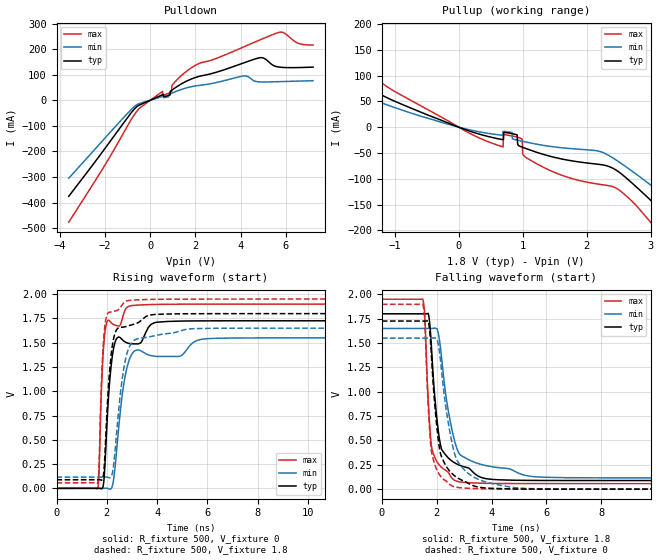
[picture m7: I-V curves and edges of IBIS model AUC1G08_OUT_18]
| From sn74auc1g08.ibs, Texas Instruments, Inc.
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[Model]   AUC1G08_OUT_18
Model_type  Output
Vref =   0
Rref =   1000
Cref =   30p
Vmeas =   0.9
| variable   typ   min   max
C_comp   7.23pF   0.09pF   19.52pF
| C_pullup   7.39pF   0.09pF   19.52pF
| C_pulldown   7.07pF   2.21pF   16.11pF
[Temperature Range]   40   100   -40
| Ambient temperature   25   85   -40
[Voltage range]   1.8   1.65   1.95
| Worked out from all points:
|   slope of the pulldown table from 0 to 0.27 V, typ, clamps not added: 25.5 ohm
|   slope of the pullup table from 0 to 0.27 V, typ, clamps not added: 23.3 ohm
|   rising waveform, R_fixture 500, V_fixture 0: 20-80 % time 284ps typ, 437ps min, 176ps max; typ from 0 V to 1.73 V
|   falling waveform, R_fixture 500, V_fixture 1.8: 20-80 % time 350ps typ, 551ps min, 215ps max; typ from 1.8 V to 0.088 V
|   rising waveform, R_fixture 500, V_fixture 1.8: 20-80 % time 274ps typ, 416ps min, 171ps max; typ from 0.088 V to 1.8 V
|   falling waveform, R_fixture 500, V_fixture 0: 20-80 % time 355ps typ, 549ps min, 221ps max; typ from 1.73 V to 0 V
[Pulldown]
| AUC1G08_OUT_18
|   Voltage   I(typ)   I(min)   I(max)
-3.6V     -375.4mA   -304.7mA   -476.5mA
-575mV    -24.07mA   -16.33mA   -41.26mA
545mV     21.87mA    15.32mA    34.57mA
550mV     22.07mA    15.45mA    18.55mA
880mV     20.93mA    25.1mA     29.42mA
950mV     39.37mA    27.68mA    32.67mA
980mV     41.16mA    28.81mA    60.67mA
1.7V      78.54mA    50.72mA    119.7mA
4.15V     146.7mA    95.14mA    209.3mA
4.85V     166.4mA    71.78mA    235.9mA
5.72V     129.6mA    72.9mA     266mA
7.2V      129.6mA    76.63mA    216.1mA
[Pullup]
| AUC1G08_OUT_18
|   Voltage   I(typ)   I(min)   I(max)
-3.6V     266.8mA    218.3mA    328.1mA
-2.79V    191.1mA    151.3mA    245.4mA
-2.285V   146mA      112.9mA    193.8mA
155mV     -7.003mA   -4.71mA    -10.82mA
945mV     -36.45mA   -25.9mA    -20.48mA
1.01V     -39.54mA   -27.72mA   -54.06mA
1.25V     -50mA      -33.78mA   -73.03mA
2.39V     -78.47mA   -58.19mA   -114.7mA
3.115V    -155.1mA   -122.9mA   -201.5mA
3.48V     -198.2mA   -157.9mA   -255.1mA
3.97V     -256.4mA   -205.8mA   -326.3mA
7.2V      -637.3mA   -526.4mA   -785.3mA
[Ramp]
| AUC1G08_OUT_18
| variable   typ   min   max
dV/dt_r   1.04/2.85E-10   0.94/4.44E-10   1.14/1.77E-10
dV/dt_f   1.03/3.53E-10   0.92/5.54E-10   1.14/2.17E-10
R_load = 500
[Rising Waveform]
| AUC1G08_OUT_18
R_fixture =   500
C_fixture =   0
L_fixture =   0
V_fixture =   0
V_fixture_min = 0
V_fixture_max = 0
|   Time   V(typ)   V(min)   V(max)
0s        6.281nV    22.82nV    528.7pV
1.63ns    88.93uV    -6.942uV   -3.924mV
1.69ns    479.5uV    -6.721uV   163mV
1.82ns    2.502mV    62.77uV    1.222V
1.955ns   389mV      706.1uV    1.662V
2.105ns   1.073V     -8.093mV   1.726V
2.29ns    1.468V     129.8mV    1.685V
2.905ns   1.492V     1.334V     1.878V
4.405ns   1.719V     1.359V     1.896V
24.99ns   1.726V     1.551V     1.898V
[Falling Waveform]
| AUC1G08_OUT_18
R_fixture =   500
C_fixture =   0
L_fixture =   0
V_fixture =   1.8
V_fixture_min = 1.65
V_fixture_max = 1.95
|   Time   V(typ)   V(min)   V(max)
0s        1.8V       1.65V      1.95V
1.495ns   1.8V       1.65V      1.949V
1.565ns   1.8V       1.65V      1.784V
1.695ns   1.802V     1.65V      893.4mV
1.82ns    1.406V     1.649V     420.4mV
2.15ns    440.3mV    1.423V     231.4mV
2.405ns   326.1mV    833.6mV    177.2mV
2.76ns    255.1mV    399.8mV    79.44mV
5.82ns    89.38mV    123.4mV    57.13mV
24.99ns   88.39mV    115.5mV    56.89mV
[Rising Waveform]
| AUC1G08_OUT_18
R_fixture =   500
C_fixture =   0
L_fixture =   0
V_fixture =   1.8
V_fixture_min = 1.65
V_fixture_max = 1.95
|   Time   V(typ)   V(min)   V(max)
0s        88.36mV    115.5mV    56.88mV
1.63ns    88.45mV    115.5mV    53.24mV
1.69ns    88.8mV     115.5mV    229.1mV
1.82ns    92.53mV    115.6mV    1.296V
1.945ns   458.5mV    116.1mV    1.717V
2.09ns    1.139V     110.4mV    1.815V
2.25ns    1.518V     198.1mV    1.821V
2.795ns   1.669V     1.382V     1.931V
5.44ns    1.799V     1.645V     1.95V
24.99ns   1.8V       1.65V      1.95V
[Falling Waveform]
| AUC1G08_OUT_18
R_fixture =   500
C_fixture =   0
L_fixture =   0
V_fixture =   0
V_fixture_min = 0
V_fixture_max = 0
|   Time   V(typ)   V(min)   V(max)
0s        1.726V     1.551V     1.898V
1.495ns   1.726V     1.551V     1.897V
1.565ns   1.726V     1.551V     1.727V
1.695ns   1.725V     1.55V      838.3mV
1.81ns    1.359V     1.55V      389.1mV
2.12ns    389.5mV    1.369V     140.9mV
2.65ns    138.1mV    367.2mV    24.44mV
3.395ns   29.47mV    117mV      6.037mV
5.105ns   1.771mV    9.413mV    492.3uV
24.99ns   24.76uV    4.693uV    11.12uV
